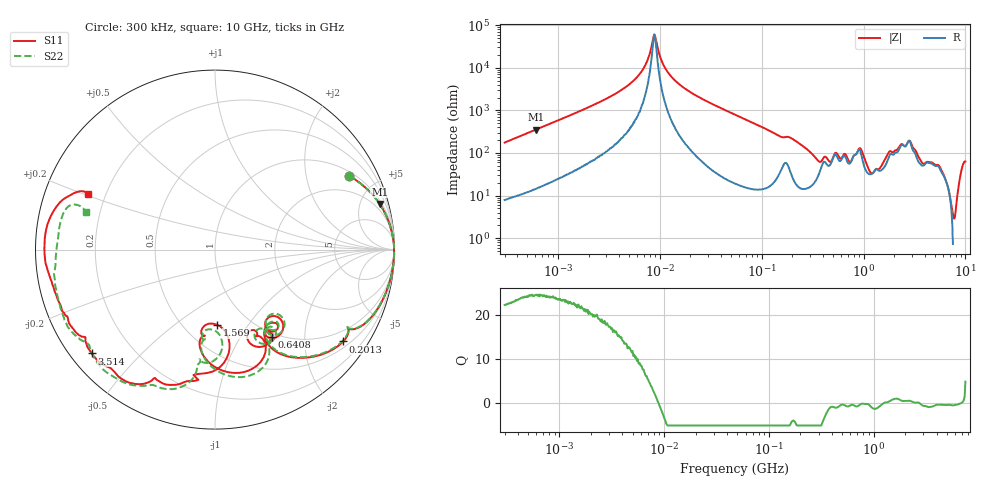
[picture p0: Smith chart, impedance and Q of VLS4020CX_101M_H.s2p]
! S-Parameter Data Generated by TDK Corporation
! Copyright(C) 2024 TDK Corporation.
! All Rights Reserved.
! TDK P/N: VLS4020CX-101M-H (SMD / SMT Inductor (Coil))
! Property: L=100uH at 1MHz
! Size(LxWxT): 4x4x2mm
! Model Type: s2p (Touchstone File Format Version 1.0)
! Frequency: DC=Yes Start=0.3MHz Stop=10000MHz 802points Log-sweep
! Model Generated on May 28, 2024
! Terms and conditions regarding TDK Simulation Models:
! 1)This simulation model is being provided solely for informational
!  purposes. Please refer to the specifications of the products in
!  terms of detailed characteristics of such products.
! 2)In no event shall TDK Corporation of any of its subsidiaries be
!  liable for any loss or damage arising, directly or indirectly,
!  from any information contained in this simulation model, including,
!  but not limited to loss or damages arising from any inaccuracies,
!  omissions or errors in connection with such information.
! 3)Any and all copyrights on this simulation model are owned by
!  TDK Corporation.  Duplication or redistribution of this simulation
!  model without prior written permission from TDK Corporation
!  is prohibited.
! 4)This simulation model is subject to any modification or change
!  without any prior notice.
! 5)Neither TDK Corporation nor any of its subsidiaries shall make any
!  warranty, express or implied, including but not limited to the
!  correctness, implied warranties of merchantability and fitness for
!  a particular purpose with respect to this simulation models.
! 6)The use of this simulation model shall be deemed to have consented
!  to the terms and conditions hereof.
! Port Assignments:
!  1 ---@@@--- 2
! Applicable Conditions:
!  Temperature = 25 degC
!  DC Bias Current = 0 A
!  Small Signal Operation
# Hz S MA R 50
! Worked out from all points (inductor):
!   801 points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, 300 kHz to 10 GHz, reference 50 ohm
!   read as one part in series: L = 92.6 uH near 318.3 kHz
!   highest Q = 24.4 at 610.3 kHz (marker M1), where L = 92.2 uH
!   self-resonance near 8.841 MHz
!   S11 on the Smith chart (normalised r, x): 300 kHz: 1.17, +3.52; 201.3 MHz: 0.66, -2.98; 640.8 MHz: 0.94, -1.38; 1.569 GHz: 0.72, -0.73; 3.514 GHz: 0.06, -0.36; 10 GHz: 0.13, +0.20
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300000  0.8524 28.9  0.4859 -58.6  0.4859 -58.6  0.8525 28.9
610333  0.9521 15.5  0.269 -72.2  0.269 -72.2  0.952 15.5
1713600  0.9905 5.5  0.09868 -81.7  0.09869 -81.7  0.9904 5.5
5784355  0.9978 0.6  0.01809 -82.9  0.01814 -83.1  0.9979 0.7
7328194  0.9982 -0.0  0.008048 -77.4  0.008015 -77.3  0.9982 -0.0
8840625  0.9983 -0.6  0.00166 -5.2  0.001689 -2.9  0.9984 -0.6
9671944  0.9984 -0.8  0.00393 65.4  0.003928 65.4  0.9985 -0.8
1.125452e7  0.9983 -1.3  0.01004 79.8  0.01007 79.9  0.9985 -1.3
1.49005e7  0.9981 -2.2  0.02246 83.8  0.02246 83.8  0.9983 -2.2
5.477226e7  0.9893 -10.6  0.1239 78.0  0.124 78.0  0.9893 -10.6
2.013356e8  0.8789 -35.6  0.3873 48.0  0.3873 48.0  0.8757 -35.0
3.126428e8  0.7014 -57.0  0.6098 24.4  0.61 24.3  0.7014 -56.4
6.407886e8  0.5783 -57.0  0.4727 -18.2  0.4728 -18.3  0.5694 -53.4
9.216398e8  0.6583 -65.7  0.3611 -26.9  0.3611 -26.9  0.71 -68.0
1.165098e9  0.5692 -97.9  0.5885 -34.1  0.5888 -34.1  0.5805 -97.1
1.569319e9  0.4192 -88.3  0.5519 -78.4  0.5523 -78.4  0.4537 -89.6
1.767019e9  0.6084 -83.8  0.3746 -97.8  0.3752 -97.9  0.609 -89.4
2.840323e9  0.8811 -122.5  0.1089 -96.1  0.1086 -96.1  0.8819 -121.1
3.514172e9  0.8974 -139.9  0.1447 -82.4  0.1447 -82.4  0.9047 -137.6
5.76861e9  0.9149 -159.3  0.09575 -105.8  0.09584 -105.9  0.925 -153.5
7.540283e9  0.9507 179.7  0.07982 -123.9  0.07988 -124.1  0.89 -175.9
1e10  0.7707 156.5  0.05795 -126.8  0.05796 -126.9  0.7455 163.9
